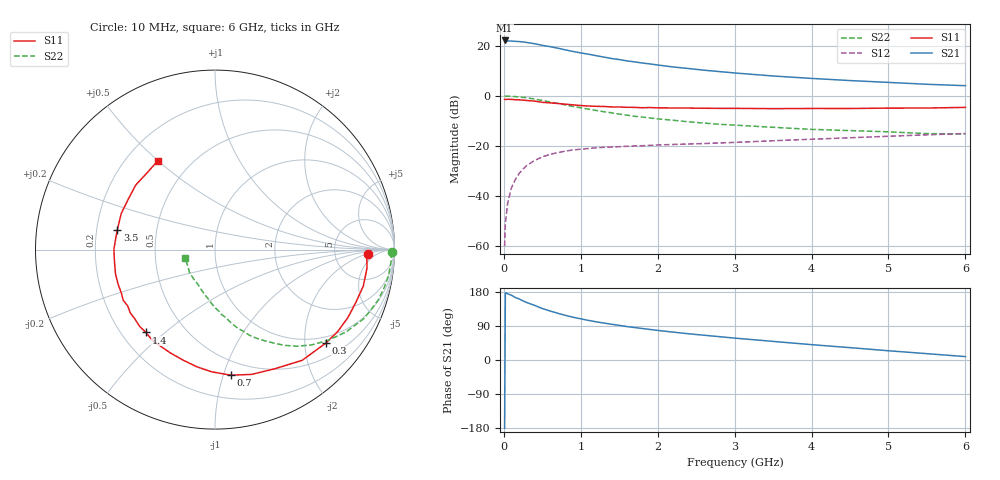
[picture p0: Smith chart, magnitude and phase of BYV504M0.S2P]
! SIEMENS Small Signal Semiconductors
! BFY420
! Si NPN RF SIEGET Grounded Emitter Transistor in MICRO-X
! VCE = 0.5 V  IC = 4 mA
! Common Emitter S-Parameters:  October  1996
# GHz  S  MA  R  50
!  f  S11  S21  S12  S22
! GHz  MAG  ANG  MAG  ANG  MAG  ANG  MAG  ANG
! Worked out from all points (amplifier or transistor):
!   36 points, 10 MHz to 6 GHz, reference 50 ohm
!   highest |S21| = 22.1 dB at 10 MHz (marker M1)
!   |S21| within 3 dB of that: start of sweep to 687.6 MHz
!   unconditionally stable (mu >= 1): 3.174 GHz to end of sweep
!   at 250 MHz: K = 0.10, MSG = 25.4 dB, |S12| = -29.2 dB
!   at 1.4 GHz: K = 0.51, MSG = 17.7 dB, |S12| = -20.4 dB
!   at 6 GHz: K = 1.21, MAG = 6.8 dB, |S12| = -15.0 dB
!   S11 on the Smith chart (normalised r, x): 10 MHz: 12, -2; 300 MHz: 0.83, -2.50; 700 MHz: 0.38, -1.06; 1.4 GHz: 0.30, -0.43; 3.5 GHz: 0.29, +0.09; 6 GHz: 0.33, +0.50
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0.01  0.8514 -1.6  12.75 -179.9  0.001 92.1  0.9857 -0.9
0.02  0.847 -2.9  12.69 177.7  0.0029 89.2  0.9834 -1.7
0.05  0.8533 -6.9  12.46 174.7  0.0073 85.7  0.9827 -4.3
0.1  0.8509 -13.8  12.42 170.7  0.0148 82.1  0.9776 -8.7
0.15  0.838 -20.6  12.23 164.9  0.0214 77.2  0.9653 -13.0
0.2  0.8317 -27.1  12.1 161.0  0.0284 75.6  0.9523 -17.0
0.25  0.8221 -33.7  11.93 155.9  0.0346 71.0  0.9319 -21.1
0.3  0.8079 -40.1  11.61 151.5  0.041 68.3  0.9132 -25.0
0.4  0.7851 -51.8  10.96 144.1  0.0513 62.0  0.8627 -32.1
0.5  0.7428 -63.4  10.19 135.8  0.0604 56.6  0.809 -38.6
0.6  0.7245 -73.7  9.599 129.4  0.068 51.3  0.7569 -44.5
0.7  0.7051 -82.9  8.949 123.4  0.0736 47.6  0.7072 -49.6
0.9  0.6605 -98.9  7.681 112.9  0.0832 40.8  0.6157 -57.8
1.1  0.627 -113.4  6.775 104.5  0.0891 36.1  0.5436 -65.1
1.4  0.6008 -129.8  5.561 94.3  0.0952 31.0  0.4593 -73.5
1.8  0.5788 -147.1  4.52 83.1  0.1012 27.0  0.377 -81.9
2.2  0.5732 -160.4  3.773 73.6  0.107 24.4  0.3259 -89.5
2.8  0.563 -176.3  3.052 61.6  0.1146 22.4  0.2704 -99.3
3.5  0.5555 168.7  2.491 49.1  0.127 20.4  0.2356 -109.1
4.5  0.5591 149.7  2.019 32.6  0.1458 16.0  0.2027 -125.3
5.5  0.5712 131.3  1.702 16.7  0.1669 10.4  0.1763 -149.8
6  0.5886 122.9  1.595 9.0  0.1771 7.2  0.174 -163.8
